FUNCTION_BLOCK Axis_PTP_Ex EXTENDS Axis_PTP IMPLEMENTS ITF_Axis, ITF_Axis_Ex
VAR_INPUT
END_VAR
VAR_OUTPUT
END_VAR
VAR
END_VAR

{warning 'add method implementation'}
METHOD M_Cyclic : BOOL
REF.ReadStatus();
Status.Axis_Ready:=REF.Status.ControlLoopClosed;
Status.Axis_Err:=REF.Status.Error;
Status.Axis_IsPTP:=REF.Status.PTPmode;
Status.Current_Pos:=REF.NcToPlc.ActPos;
END_METHOD

METHOD M_Home : BOOL
VAR_INPUT
	Execute:BOOL;
END_VAR
VAR_STAT
	mcHome:Tc2_MC2.MC_Home;
END_VAR
mcHome(
	Axis:= REF, 
	Execute:= Execute, 
	Position:= PARA.RefPos,
	bCalibrationCam:= DrvIn.HomeSensor);
END_METHOD

METHOD M_Reset : BOOL
VAR_INPUT
	Execute:BOOL;
END_VAR
VAR_STAT
	mcReset:Tc2_MC2.MC_Reset;
END_VAR
mcReset(
	Axis:=REF , 
	Execute:=EXECUTE);
END_METHOD

END_FUNCTION_BLOCK
